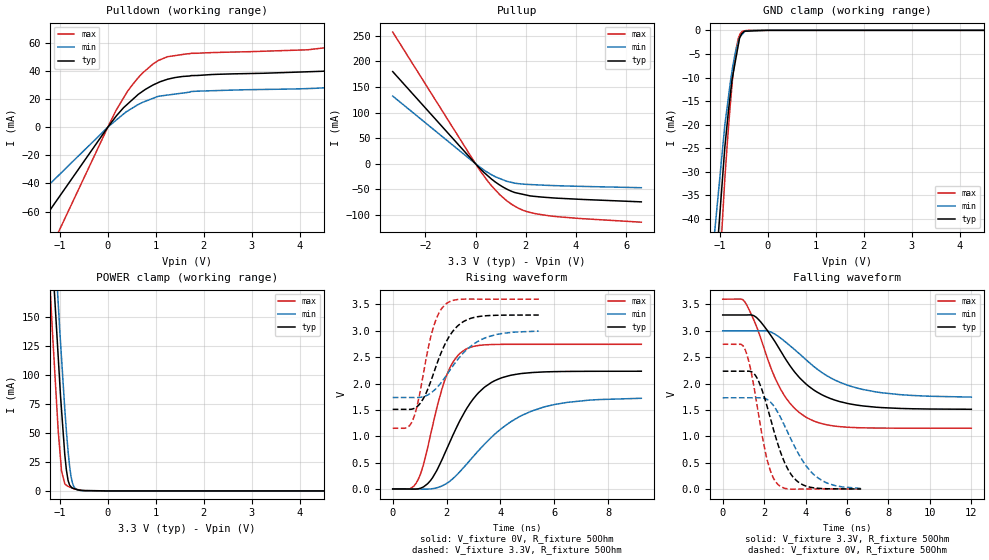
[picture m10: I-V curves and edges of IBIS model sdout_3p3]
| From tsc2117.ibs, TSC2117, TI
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|   sdout_3p3 Model
[Model]   sdout_3p3
Model_type   3-state
Polarity   Non-Inverting
Vmeas = 1.65
Vref = 1.65
Cref = 10pF
Rref = 50
|   typ   min   max
|   (nom PVT)   (fast PVT)   (slow PVT)
|C_comp from frequency sweep method (F=25MHz)
|C_comp   4.219e-12   3.842e-12   4.514e-12
|ON state : BUFFER OUTPUT TURNED HIGH
|C_comp   4.219e-12   3.842e-12   4.514e-12
|OFF state: BUFFER IN HIGH IMPEDANCE
|C_comp   1.606e-12   1.601e-12   1.607e-12
|C_comp from LC tank measurement(L=1nH)
|Resonant Frequency(Hz)   4.010e+09   4.070e+09   3.940e+09
C_comp   1.577e-12   1.531e-12   1.633e-12
|ON state : BUFFER OUTPUT TURNED HIGH
|Resonant Frequency(Hz)   4.010e+09   4.070e+09   3.940e+09
|C_comp   1.577e-12   1.531e-12   1.633e-12
|OFF state: BUFFER IN HIGH IMPEDANCE
|Resonant Frequency(Hz)   4.390e+09   4.410e+09   4.380e+09
|C_comp   1.316e-12   1.304e-12   1.322e-12
| Where nom  PVT is Nominal Process, 3.3V, 48C
|   Fast PVT is Strong Process,  3.6V, -40C
|   Slow PVT is Weak Process,   3V, 108C
[Voltage Range]   3.3   3   3.6
|Ambient Temperature   25   85   -40
|Junction Temperature
[Temperature Range]   48   108   -40
[Pullup Reference]   3.3   3   3.6
[Pulldown Reference]   0   0   0
[Power Clamp Reference]   3.3   3   3.6
[GND Clamp Reference]   0   0   0
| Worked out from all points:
|   slope of the pulldown table from 0 to 0.495 V, typ, clamps not added: 26.1 ohm
|   slope of the pullup table from 0 to 0.495 V, typ, clamps not added: 20.8 ohm
|   GND clamp passes 1 mA (typ) near -0.56 V on its own axis
|   POWER clamp passes 1 mA (typ) near -0.63 V on its own axis
|   falling waveform, V_fixture 3.3V, R_fixture 50Ohm: 20-80 % time 2.16ns typ, 2.7ns min, 1.61ns max; typ from 3.3 V to 1.51 V
|   rising waveform, V_fixture 0V, R_fixture 50Ohm: 20-80 % time 1.39ns typ, 2.2ns min, 849ps max; typ from 0 V to 2.23 V
|   rising waveform, V_fixture 3.3V, R_fixture 50Ohm: 20-80 % time 881ps typ, 1.24ns min, 601ps max; typ from 1.51 V to 3.3 V
|   falling waveform, V_fixture 0V, R_fixture 50Ohm: 20-80 % time 1.08ns typ, 1.45ns min, 763ps max; typ from 2.23 V to 0 V
[Pulldown]
|   Voltage   I(typ)   I(min)   I(max)
-3.3V     -161.2mA   -110.2mA   -239mA
-3mV      -146.6uA   -100.2uA   -217.3uA
172.8mV   7.814mA    4.962mA    12.02mA
478.8mV   18.5mA     12.87mA    28.66mA
720mV     25.34mA    17.58mA    38.31mA
1.062V    31.82mA    21.98mA    47.5mA
1.735V    36.63mA    25.3mA     52.44mA
4.162V    39.33mA    27.4mA     54.94mA
4.507V    39.8mA     27.95mA    56.32mA
5.148V    43.41mA    30.52mA    62.67mA
5.67V     50.21mA    35.31mA    74.15mA
6.6V      76.92mA    49.15mA    118mA
[GND Clamp]
|   Voltage   I(typ)   I(min)   I(max)
-3.3V     -1.747A    -1.57A     -1.979A
-1.512V   -108.8mA   -85.88mA   -141.2mA
-897.6mV  -24.89mA   -20.19mA   -31.57mA
-784.8mV  -13.83mA   -11.26mA   -15.95mA
-745.8mV  -10.4mA    -8.578mA   -11.48mA
-694.8mV  -7.537mA   -5.639mA   -6.486mA
-655.2mV  -5.318mA   -3.843mA   -3.618mA
-619.2mV  -3.3mA     -2.569mA   -1.849mA
-590.7mV  -1.702mA   -1.563mA   -1.046mA
-529.2mV  -577.9uA   -784uA     -189.3uA
-285mV    -109.3uA   -1.799uA   -4.76uA
6.6V      0A         0A         0A
[Pullup]
|   Voltage   I(typ)   I(min)   I(max)
-3.3V     180mA      132.2mA    257.1mA
172.8mV   -9.066mA   -6.319mA   -12.96mA
633.6mV   -29.81mA   -21.35mA   -42.9mA
939.6mV   -40.79mA   -28.36mA   -59.08mA
1.246V    -49.52mA   -34.23mA   -72.34mA
1.554V    -56.04mA   -37.69mA   -82.56mA
1.904V    -59.8mA    -39.73mA   -91.02mA
2.473V    -64.21mA   -41.21mA   -98.18mA
4.162V    -69.36mA   -44.01mA   -106.8mA
6.6V      -74.32mA   -46.7mA    -114mA
[POWER Clamp]
|   Voltage   I(typ)   I(min)   I(max)
-3.3V     1.978A     1.996A     1.965A
-1.3V     314.4mA    363.1mA    252.8mA
-1.156V   203.5mA    250.7mA    138.1mA
-1.112V   170.3mA    218.3mA    107.1mA
-1.037V   117.4mA    163.9mA    53.48mA
-964.8mV  69.74mA    114.5mA    17.03mA
-897.6mV  31.4mA     70.73mA    6.18mA
-864.6mV  18.26mA    52.05mA    5.001mA
-825mV    8.486mA    32.44mA    3.888mA
-771mV    3.758mA    13.46mA    2.968mA
-694.8mV  1.854mA    2.979mA    1.671mA
6.6V      0A         0A         0A
[Ramp]
R_load = 50
|   typ   min   max
dV/dt_r   1.34028/1.38772e-09   1.03716/2.22033e-09   1.64702/8.45795e-10
dV/dt_f   1.07315/2.15827e-09   0.754572/2.69104e-09   1.46873/1.61283e-09
[Falling Waveform]
V_fixture = 3.3V
V_fixture_min = 3V
V_fixture_max = 3.6V
R_fixture = 50Ohm
|   Time   V(typ)   V(min)   V(max)
0s        3.3V       3V         3.6V
1.062ns   3.3V       3V         3.551V
1.661ns   3.241V     3V         3.053V
2.337ns   2.904V     2.974V     2.285V
2.773ns   2.633V     2.869V     1.908V
3.402ns   2.254V     2.666V     1.557V
4.132ns   1.954V     2.412V     1.337V
5.419ns   1.685V     2.065V     1.192V
6.753ns   1.575V     1.888V     1.16V
12ns      1.511V     1.742V     1.152V
[Rising Waveform]
V_fixture = 0V
V_fixture_min = 0V
V_fixture_max = 0V
R_fixture = 50Ohm
|   Time   V(typ)   V(min)   V(max)
0s        2.454nV    8.214nV    904.1pV
645ps     -788.1uV   -4.802uV   4.262mV
925ps     973.8uV    -341.8uV   159.1mV
1.412ns   166.3mV    1.386mV    1.045V
1.973ns   721.1mV    95.92mV    2.118V
2.309ns   1.101V     231.9mV    2.461V
2.686ns   1.475V     437.2mV    2.643V
3.669ns   2.022V     983.1mV    2.74V
5.164ns   2.209V     1.479V     2.745V
9.23ns    2.234V     1.72V      2.745V
[Rising Waveform]
V_fixture = 3.3V
V_fixture_min = 3V
V_fixture_max = 3.6V
R_fixture = 50Ohm
|   Time   V(typ)   V(min)   V(max)
0s        1.51V      1.735V     1.152V
514ps     1.51V      1.735V     1.159V
730ps     1.517V     1.735V     1.29V
933ps     1.575V     1.735V     1.636V
1.127ns   1.707V     1.75V      2.15V
1.477ns   2.134V     1.844V     3.01V
1.985ns   2.791V     2.149V     3.515V
2.594ns   3.166V     2.564V     3.6V
3.285ns   3.278V     2.833V     3.601V
5.424ns   3.3V       2.995V     3.6V
[Falling Waveform]
V_fixture = 0V
V_fixture_min = 0V
V_fixture_max = 0V
R_fixture = 50Ohm
|   Time   V(typ)   V(min)   V(max)
0s        2.234V     1.73V      2.745V
1.092ns   2.234V     1.73V      2.634V
1.579ns   2.154V     1.73V      1.777V
2.099ns   1.625V     1.708V     627.5mV
2.37ns    1.245V     1.621V     274.4mV
2.675ns   834.8mV    1.441V     81.48mV
3.392ns   227.4mV    865.6mV    -3.469mV
4.361ns   23.15mV    286.2mV    -219.8uV
5.12ns    3.19mV     99.39mV    102.9uV
6.683ns   160.3uV    9.803mV    7.569uV
